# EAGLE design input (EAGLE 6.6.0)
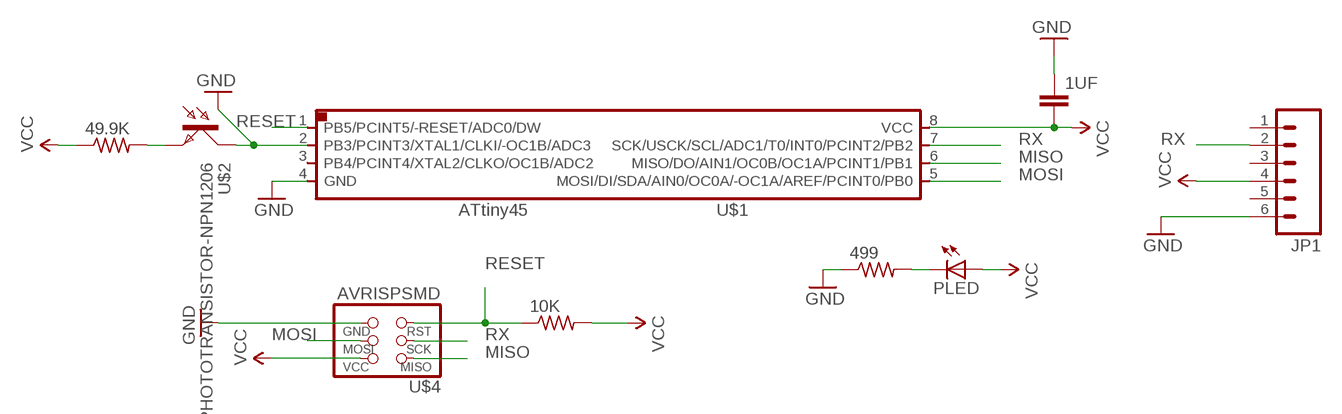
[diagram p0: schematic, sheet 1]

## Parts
1UF  CAP1206  [1206]
10K  RESISTOR1206  [1206]
49.9K  RESISTOR1206  [1206]
499  RESISTOR1206  [1206]
JP1  M06SMD  [1X06-SMD]
PLED  LED1206  [1206]
U$1  ATTINY45SI  [SOIC8]
U$2  PHOTOTRANSISTOR-NPN1206  [OP1206]
U$4  AVRISPSMD  [2X03SMD]

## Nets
GND: 1UF.1 499.1 JP1.6 U$1.2(PB3/PCINT3/XTAL1/CLKI/-OC1B/ADC3) U$1.4(GND) U$2.COLLECTOR(C) U$4.6(GND)
MISO: U$1.6(MISO/DO/AIN1/OC0B/OC1A/PCINT1/PB1) U$4.1(MISO)
MOSI: U$1.5(MOSI/DI/SDA/AIN0/OC0A/-OC1A/AREF/PCINT0/PB0) U$4.4(MOSI)
N$1: 49.9K.2 U$2.EMITTER(E)
N$2: 499.2 PLED.2(C)
RESET: 10K.1 U$1.1(PB5/PCINT5/-RESET/ADC0/DW) U$4.5(RST)
RX: JP1.2 U$1.7(SCK/USCK/SCL/ADC1/T0/INT0/PCINT2/PB2) U$4.3(SCK)
VCC: 1UF.2 10K.2 49.9K.1 JP1.4 PLED.1(A) U$1.8(VCC) U$4.2(VCC)
Unconnected: JP1.1 JP1.3 JP1.5 U$1.3(PB4/PCINT4/XTAL2/CLKO/OC1B/ADC2)

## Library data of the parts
1UF = 01_SparkFun:CAP: Capacitor
10K 49.9K 499 = ng:RESISTOR
JP1 = 01_SparkFun:M06: Header 6 Standard 6-pin 0.1" header. Use with straight break away headers (SKU : PRT-00116), right angle break away headers (PRT-00553), swiss pins (PRT-00743), machine pins (PRT-00117), and female headers (PRT-00115). Molex polarized connector foot print use with SKU : PRT-08094 with associated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
PLED = 01_ng:LED
U$1 = 01_fab:ATTINY45
U$2 = 01_fab:PHOTOTRANSISTOR-NPN
U$4 = fab:AVRISP

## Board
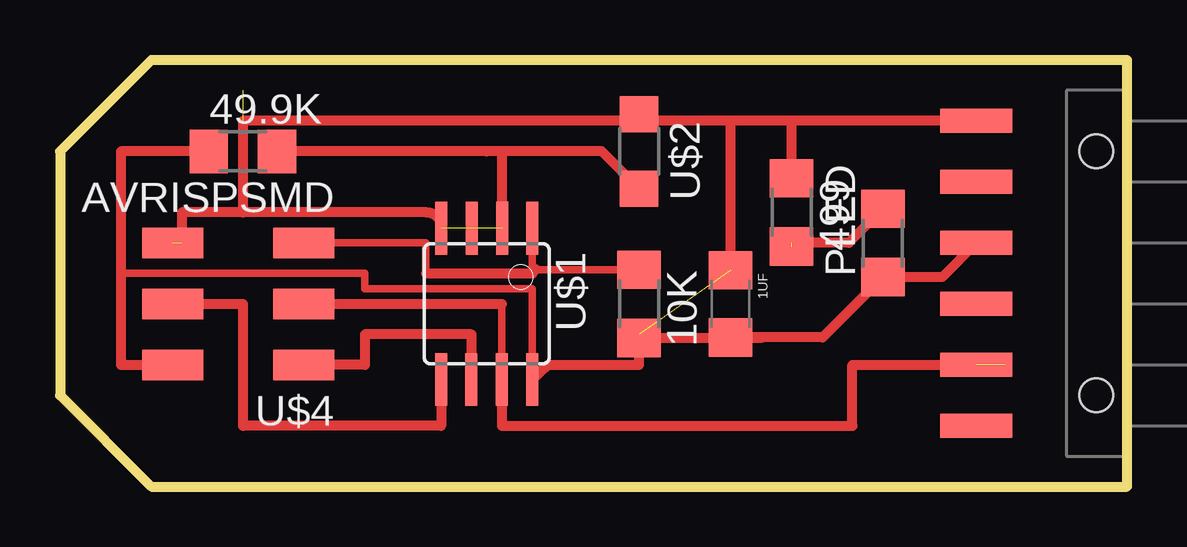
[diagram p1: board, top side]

Size 44.45 x 17.78 mm. Coordinates in mm from the lower left corner, seen from the top.
Outline: 44.45,17.78 3.81,17.78 0,13.97 0,3.81 3.81,0 44.45,0 44.45,17.78
Copper layers (1*16): Top 0.035mm / dielectric 1.5mm / Bottom 0.035mm
Design rules "default": minimum track width 10mil, minimum drill 24mil, track to track 8mil, track to pad 8mil, pad to pad 8mil, via to via 8mil, smd to smd 8mil, copper to edge 40mil, drill to drill 8mil, minimum pad ring 10mil, minimum via ring 8mil, stop-mask expansion 4mil, vias tented up to drill 0mil, thermal gap 10mil

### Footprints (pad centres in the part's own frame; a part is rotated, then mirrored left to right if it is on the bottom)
1206 = smd 1.6 x 1.8: 1 -1.4,0; 2 1.4,0
1206' = smd 1.6 x 1.803: 1 -1.422,0; 2 1.422,0
1X06-SMD = smd 1 x 3: 1 -6.35,5; 2 -3.81,5; 3 -1.27,5; 4 1.27,5; 5 3.81,5; 6 6.35,5 | hole 1.4: -5.08,0; 5.08,0
SOIC8 = smd 0.5 x 2.2: 1 -1.905,-3.154; 2 -0.645,-3.154; 3 0.625,-3.154; 4 1.895,-3.154; 5 1.905,3.154; 6 0.635,3.154; 7 -0.635,3.154; 8 -1.905,3.154
OP1206 = smd 1.5 x 1.6: COLLECTOR -1.55,0; EMITTER 1.55,0
2X03SMD = smd 2.54 x 1.27: 1 -2.54,2.54; 2 2.92,2.54; 3 -2.54,0; 4 2.92,0; 5 -2.54,-2.54; 6 2.92,-2.54

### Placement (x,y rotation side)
1UF  27.94,7.62 270 top
10K  [1206']  24.13,7.62 270 top
49.9K  [1206']  7.62,13.97 0 top
499  [1206']  30.48,11.43 270 top
JP1  43.18,8.89 90 top
PLED  [1206']  34.29,10.16 90 top
U$1  17.78,7.62 180 top
U$2  24.13,13.97 270 top
U$4  7.62,7.62 180 top

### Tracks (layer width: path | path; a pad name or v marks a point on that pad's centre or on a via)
GND  (4 unrouted)
  Top 0.406: JP1.6 30.48,15.24 | 30.48,15.24 27.94,15.24 | 27.94,15.24 24.13,15.24 | 24.13,15.24 U$2.COLLECTOR | 24.13,6.22 24.13,6.35 | 1UF.1 27.94,15.24 | 499.1 30.48,15.24 | 7.62,11.43 15.27,11.43 arc-90 15.88,10.82 U$1.4 | 7.62,11.43 5.08,11.43 5.08,10.16 | 7.62,11.43 7.62,15.24 24.13,15.24 | U$1.2 18.43,13.97 17.78,13.97
MISO
  Top 0.406: U$1.6 17.15,6.35 12.7,6.35 12.7,5.08 U$4.1
MOSI
  Top 0.406: U$4.4 7.62,7.62 7.62,2.54 15.88,2.54 U$1.5
N$1
  Top 0.406: U$2.EMITTER 22.58,13.97 49.9K.2
N$2  (1 unrouted)
  Top 0.406: PLED.2 32.87,10.16 30.48,10.16
RESET
  Top 0.305: 19.68,8.89 U$1.1 | U$4.5 15.24,10.16 15.24,8.89 | 19.84,9.04 10K.1
  Top 0.406: 15.24,8.89 19.68,8.89 arc-90 19.84,9.04
RX  (1 unrouted)
  Top 0.305: 18.41,7.62 U$1.7
  Top 0.406: U$4.3 18.41,7.62 | U$1.7 18.41,2.54 33.02,2.54 33.02,5.08 39.37,5.08
VCC
  Top 0.305: U$1.8 19.68,8.25 12.7,8.25 12.7,8.89 2.54,8.89
  Top 0.406: JP1.4 36.76,8.74 PLED.1 31.77,6.22 29.21,6.22 | 29.21,6.22 1UF.2 | 29.21,6.22 29.21,6.2 10K.2 24.13,5.08 20.34,5.08 U$1.8 | U$4.2 2.54,5.08 2.54,8.89 2.54,13.97 49.9K.1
